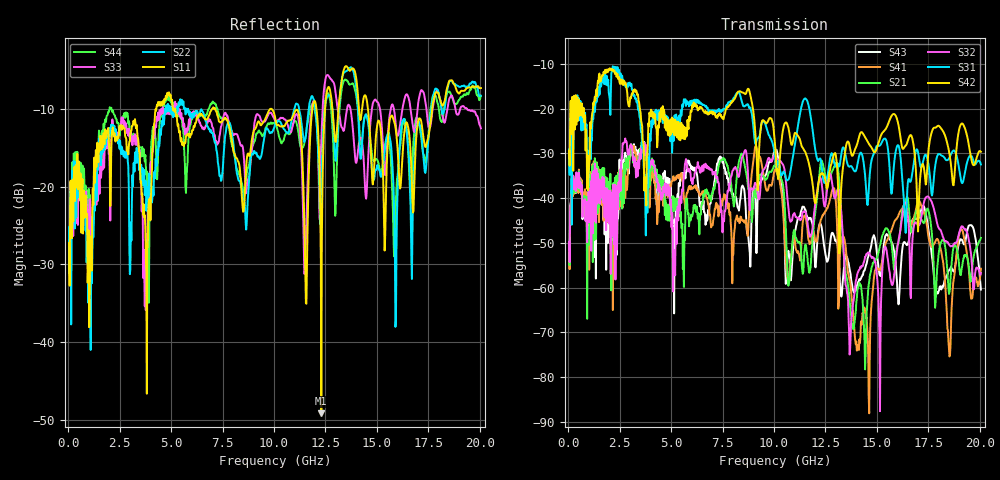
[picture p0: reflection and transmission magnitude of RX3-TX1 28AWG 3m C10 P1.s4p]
! FILE: O:\PROJECTS\SI-2007-05-003 3m Eyemax Qual\XT\FD\RX3-TX1 28AWG 3m C10 P1.s4p
# MHZ S RI R 50.00
! FREQ  S11  S12  S13  S14
!  S21  S22  S23  S24
!  S31  S32  S33  S34
!  S41  S42  S43  S44
!  REAL  IMAG  REAL  IMAG  REAL  IMAG  REAL  IMAG
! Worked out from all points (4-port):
!   801 points, 50 MHz to 20.05 GHz, reference 50 ohm
!   strongest paths, dB at 50 MHz, 5.05 GHz, 10.05 GHz, 15.05 GHz, 20.05 GHz:
!     S42: -29.4, -22.0, -27.9, -28.1, -29.6
!     S31: -29.1, -29.9, -30.5, -28.3, -32.5
!     S32: -49.8, -43.3, -30.4, -60.3, -56.7
!     S21: -51.0, -40.8, -32.8, -52.6, -48.9
!     S41: -51.6, -36.2, -33.7, -56.0, -55.8
!     S43: -51.1, -40.1, -29.3, -54.5, -60.4
!   lowest |S11| = -49.2 dB at 12.3 GHz (marker M1), VSWR 1.01, Z = 50.1 - j0.333 ohm
!   |S11| at or under -10 dB: start of sweep to 4.285 GHz; 7.148 GHz to 9.818 GHz (2.67 GHz wide, 31.5 % of centre); 14.56 GHz to 17.69 GHz (3.121 GHz wide, 19.4 % of centre)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
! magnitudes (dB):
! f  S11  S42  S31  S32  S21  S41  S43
! 50 MHz  -27.2  -29.4  -29.1  -49.8  -51.0  -51.6  -51.1
! 9.125 GHz  -12.4  -27.6  -27.8  -36.8  -39.6  -28.3  -44.6
! 10.72 GHz  -11.5  -24.8  -35.7  -43.5  -58.9  -57.7  -52.4
! 12.3 GHz  -49.2  -34.5  -32.3  -36.1  -31.7  -44.7  -46.2
! 14.43 GHz  -8.2  -26.4  -34.9  -53.1  -78.3  -65.1  -55.8
! 16.4 GHz  -11.8  -28.2  -47.8  -41.1  -40.7  -44.8  -50.2
! 20.05 GHz  -7.3  -29.6  -32.5  -56.7  -48.9  -55.8  -60.4
